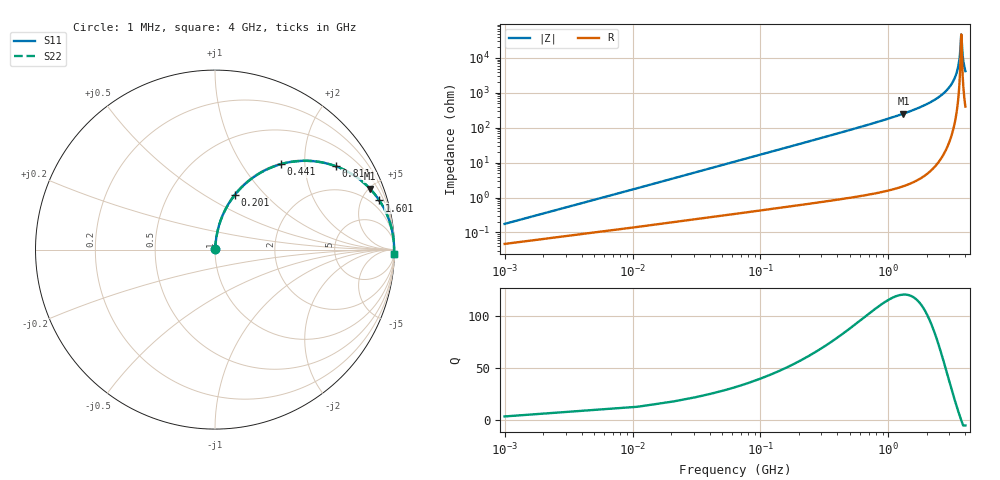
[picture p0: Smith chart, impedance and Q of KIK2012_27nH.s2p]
!version-2
!date-01.2022
!Series
# MHz S RI R 50
!Freq ReS11 ImS11 ReS21 ImS21 ReS12 ImS12 ReS22 ImS22
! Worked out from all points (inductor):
!   401 points, 1 MHz to 4 GHz, reference 50 ohm
!   read as one part in series: L = 27 nH near 21 MHz
!   highest Q = 120 at 1.311 GHz (marker M1), where L = 30.8 nH
!   self-resonance near 3.711 GHz
!   S11 on the Smith chart (normalised r, x): 1 MHz: 1.00, +0.00; 201 MHz: 1.01, +0.68; 441 MHz: 1.02, +1.52; 811 MHz: 1.03, +2.89; 1.601 GHz: 1.06, +6.67; 4 GHz: 9, -84
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1  0.000472 0.00169  0.9995 -0.00169  0.9995 -0.00169  0.000472 0.00169
31  0.00513 0.0522  0.9949 -0.0522  0.9949 -0.0522  0.00513 0.0522
51  0.0104 0.0854  0.9896 -0.0854  0.9896 -0.0854  0.0104 0.0854
111  0.0383 0.1804  0.9617 -0.1804  0.9617 -0.1804  0.0383 0.1804
201  0.109 0.3029  0.891 -0.3029  0.891 -0.3029  0.109 0.3029
441  0.367 0.476  0.633 -0.476  0.633 -0.476  0.367 0.476
671  0.5799 0.4886  0.4201 -0.4886  0.4201 -0.4886  0.5799 0.4886
811  0.6746 0.4639  0.3254 -0.4639  0.3254 -0.4639  0.6746 0.4639
1311  0.8638 0.3388  0.1362 -0.3388  0.1362 -0.3388  0.8638 0.3388
1341  0.8705 0.3316  0.1295 -0.3316  0.1295 -0.3316  0.8705 0.3316
1601  0.9156 0.2737  0.0844 -0.2737  0.0844 -0.2737  0.9156 0.2737
2001  0.9563 0.1995  0.0437 -0.1995  0.0437 -0.1995  0.9563 0.1995
2671  0.987 0.1049  0.013 -0.1049  0.013 -0.1049  0.987 0.1049
3061  0.9944 0.0612  0.00563 -0.0612  0.00563 -0.0612  0.9944 0.0612
3341  0.9969 0.0334  0.00306 -0.0334  0.00306 -0.0334  0.9969 0.0334
3571  0.9978 0.0123  0.00219 -0.0123  0.00219 -0.0123  0.9978 0.0123
3631  0.9979 0.00705  0.00212 -0.00705  0.00212 -0.00705  0.9979 0.00705
3711  0.9979 0.000157  0.00211 -0.000157  0.00211 -0.000157  0.9979 0.000157
3731  0.9979 -0.00154  0.00212 0.00154  0.00212 0.00154  0.9979 -0.00154
3781  0.9978 -0.00575  0.00218 0.00575  0.00218 0.00575  0.9978 -0.00575
3831  0.9977 -0.0099  0.00227 0.0099  0.00227 0.0099  0.9977 -0.0099
4000  0.9972 -0.0236  0.00283 0.0236  0.00283 0.0236  0.9972 -0.0236
